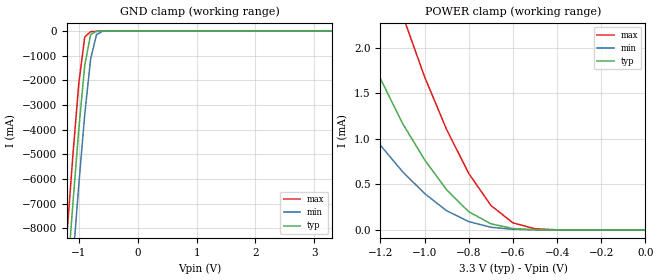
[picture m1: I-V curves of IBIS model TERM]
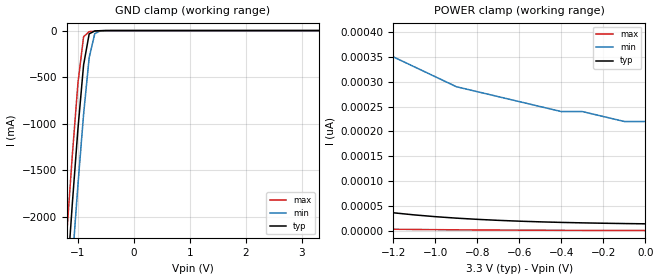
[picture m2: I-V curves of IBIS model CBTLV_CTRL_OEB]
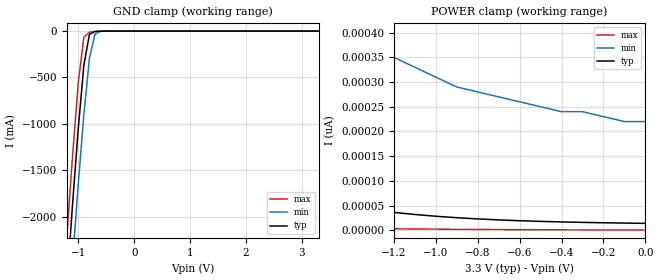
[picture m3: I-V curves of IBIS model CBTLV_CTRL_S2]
| I/O Buffer Information Specification (IBIS) Version 3.2 (August 20, 1999)
| IBIS is a standard for electronic behavioral specifications of integrated
| circuit input/output analog characteristics.
[IBIS Ver]   3.2
[File Name]   cbtlv3251.ibs
[File Rev]   1.1
[Date]   Tuesday, October 16 2001
[Source]   Integrated Device Technology, Inc.
[Notes]   1.Temperatures: typ=25C, min=-40C, max=100C
[Disclaimer] Integrated Device Technology, Inc. ("IDT") hereby grants the
   user of this IBIS model a non-exclusive, nontransferable
   license to use this IBIS model under the following terms. The
   user is granted this license only to use the IBIS model and is
   not granted rights to sell, copy (except as needed to run the
   IBIS model), rent, lease or sub-license the IBIS model in
   whole or in part, or in modified form to anyone. The User may
   modify the IBIS model to suit its specific applications, but
   rights to derivative works and such modifications shall belong
   to IDT.
   This IBIS model is provided on an AS IS" basis and IDT
   makes absolutely no warranty with respect to the information
   contained herein. IDT DISCLAIMS AND CUSTOMER WAIVES ALL
   WARRANTIES, EXPRESS AND IMPLIED, INCLUDING WARRANTIES OF
   MERCHANTABILITY AND FITNESS FOR A PARTICULAR PURPOSE. THE
   ENTIRE RISK AS TO QUALITY AND PERFORMANCE IS WITH THE USER
   ACCORDINGLY, IN NO EVENT SHALL IDT BE LIABLE FOR ANY DIRECT OR
   INDIRECT DAMAGES, WHETHER IN CONTRACT OR TORT,  INCLUDING
   ANY LOST PROFITS OR OTHER INCIDENTAL, CONSEQUENTIAL, EXEMPLARY,
   OR PUNITIVE DAMAGES ARISING OUT OF THE USE OR APPLICATION OF
   THE IBIS model.
   Further, IDT reserves the right to make changes without notice
   to any product herein to improve reliability, function, or
   design. IDT does not convey any license under patent rights or
   any other intellectual property rights, including those of
   third parties. IDT is not obligated to provide maintenance or
   support for the licensed IBIS model.
[Copyright]   Copyright 1997, Integrated Device Technology, Inc. all rights
   reserved
|   Component IDT74CBTLV3251
[Component]   IDT74CBTLV3251
[Manufacturer]   Integrated Device Technology
[Package]
|Following package parameters are for SSOP 16 lead package
| variable   typ   min   max
R_pkg   9.80m   9.60m   10.20m
L_pkg   2.30nH   2.00nH   2.90nH
C_pkg   0.12pF   0.10pF   0.13pF
[Pin]  signal_name   model_name   R_pin   L_pin   C_pin
1   B4   TERM
2   B3   TERM
3   B2   TERM
4   B1   TERM
5   A   TERM
6   NC   TERM
7   _OE_   CBTLV_CTRL_OEB
8   GND   GND
9   S2   CBTLV_CTRL_S2
10   S1   CBTLV_CTRL_S1
11   S0   CBTLV_CTRL_S0
12   B8   TERM
13   B7   TERM
14   B6   TERM
15   B5   TERM
16   VCC   POWER
| oeb  oeb   dummy_model
[Series Switch Groups]
|Function Group States
On A /
On B /
On C /
On D /
On E /
On F /
On G /
On H /
Off A B C D E F G H /
[Series Pin Mapping]   pin_2   model_name   function_table_group
5   1   CBTLV_SW   A
5   2   CBTLV_SW   B
5   3   CBTLV_SW   C
5   4   CBTLV_SW   D
5   12   CBTLV_SW   E
5   13   CBTLV_SW   F
5   14   CBTLV_SW   G
5   15   CBTLV_SW   H
|   Model CBTLV_SW
[Model]   CBTLV_SW
Model_type   Series_switch
C_comp   0.00pF   0.00pF   0.00pF
[Temperature Range]   25.00   100.00   -40.00
[Voltage Range]   3.30V   3.00V   3.6V
[On]
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[Off]
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| Models and submodels in the file (6): TERM (Terminator), CBTLV_CTRL_OEB (Input), CBTLV_CTRL_S0 (Input), CBTLV_CTRL_S1 (Input), CBTLV_CTRL_S2 (Input), CBTLV_SW (Series_switch)
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|   Model TERM
[Model]   TERM
Model_type   Terminator
Polarity   Non-Inverting
C_comp   5.00pF   5.00pF   5.00pF
[Temperature Range]   25.00   100.00   -40.00
[Voltage Range]   3.30V   3.00V   3.60V
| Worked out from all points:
|   GND clamp passes 1 mA (typ) near -0.54 V on its own axis
|   POWER clamp passes 1 mA (typ) near -1.06 V on its own axis
[GND_clamp]
| voltage   I(typ)   I(min)   I(max)
-3.3V     -82.19A    -84.14A    -80.6A
-1.2V     -10.13A    -12.44A    -8.17A
-1.1V     -6.95A     -9.26A     -5A
-1V       -3.95A     -6.2A      -2.1A
-900mV    -1.39A     -3.38A     -240mA
-800mV    -140mA     -1.13A     -23mA
-700mV    -10.38mA   -140mA     -11.02mA
-600mV    -2.14mA    -10.9mA    -3.97mA
3.3V      43.59pA    38.63nA    59.54pA
[POWER_clamp]
| voltage   I(typ)   I(min)   I(max)
-3.3V     19.83mA    14.03mA    24.7mA
-1.6V     4.15mA     2.52mA     6.59mA
-1.5V     3.45mA     2.06mA     5.66mA
-1.3V     2.2mA      1.26mA     3.9mA
-1.1V     1.17mA     640uA      2.36mA
-1V       770uA      400uA      1.68mA
-900mV    440uA      210uA      1.1mA
-800mV    200uA      91.79uA    620uA
-700mV    67.88uA    29.64uA    270uA
-600mV    15.52uA    7.26uA     77.81uA
-500mV    2.7uA      1.47uA     13.43uA
0V        43.57pA    640pA      91.39pA
|   Model CBTLV_CTRL_OEB
[Model]   CBTLV_CTRL_OEB
Model_type   Input
Vinl =   0.80V
Vinh =   2.00V
C_comp   5.00pF   5.00pF   5.00pF
[Temperature Range]   25.00   100.00   -40.00
[Voltage Range]   3.30V   3.00V   3.60V
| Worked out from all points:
|   GND clamp passes 1 mA (typ) near -0.58 V on its own axis
[GND_clamp]
| voltage   I(typ)   I(min)   I(max)
-3.3V     -21.99A    -22.53A    -21.55A
-1.2V     -2.71A     -3.32A     -2.18A
-1.1V     -1.85A     -2.47A     -1.33A
-1V       -1.05A     -1.65A     -560mA
-900mV    -370mA     -900mA     -66.57mA
-800mV    -35.21mA   -290mA     -11.53mA
-700mV    -4.04mA    -32.91mA   -5.99mA
-600mV    -1.16mA    -2.33mA    -2.18mA
3.3V      14.09pA    240pA      630fA
[POWER_clamp]
| voltage   I(typ)   I(min)   I(max)
-3.3V     620pA      3.78nA     60.87pA
-3V       430pA      2.65nA     42.45pA
-2.9V     380pA      2.34nA     37.47pA
-2.6V     260pA      1.61nA     25.42pA
-2.3V     170pA      1.1nA      16.83pA
-2V       110pA      760pA      10.91pA
-1.8V     83.99pA    610pA      8.08pA
-1.4V     47.41pA    410pA      4.34pA
-1.2V     36.3pA     350pA      3.17pA
-900mV    25.54pA    290pA      2.02pA
-400mV    16.95pA    240pA      1.06pA
0V        14.1pA     220pA      740fA
|   Model CBTLV_CTRL_S2
[Model]   CBTLV_CTRL_S2
Model_type   Input
Vinl =   0.80V
Vinh =   2.00V
C_comp   5.00pF   5.00pF   5.00pF
[Temperature Range]   25.00   100.00   -40.00
[Voltage Range]   3.30V   3.00V   3.60V
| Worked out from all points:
|   GND clamp passes 1 mA (typ) near -0.58 V on its own axis
[GND_clamp]
| voltage   I(typ)   I(min)   I(max)
-3.3V     -22A       -22.54A    -21.56A
-1.2V     -2.71A     -3.33A     -2.18A
-1.1V     -1.85A     -2.47A     -1.33A
-1V       -1.05A     -1.65A     -560mA
-900mV    -370mA     -900mA     -66.52mA
-800mV    -35.18mA   -290mA     -11.47mA
-700mV    -4.02mA    -32.89mA   -5.96mA
-600mV    -1.16mA    -2.31mA    -2.17mA
3.3V      14.11pA    240pA      630fA
[POWER_clamp]
| voltage   I(typ)   I(min)   I(max)
-3.3V     620pA      3.78nA     60.89pA
-3V       430pA      2.65nA     42.48pA
-2.9V     380pA      2.34nA     37.5pA
-2.6V     260pA      1.61nA     25.42pA
-2.3V     170pA      1.1nA      16.85pA
-2V       110pA      760pA      10.91pA
-1.8V     84.03pA    610pA      8.09pA
-1.4V     47.41pA    410pA      4.34pA
-1.2V     36.31pA    350pA      3.19pA
-900mV    25.54pA    290pA      2.02pA
-400mV    16.97pA    240pA      1.06pA
0V        14.1pA     220pA      750fA
